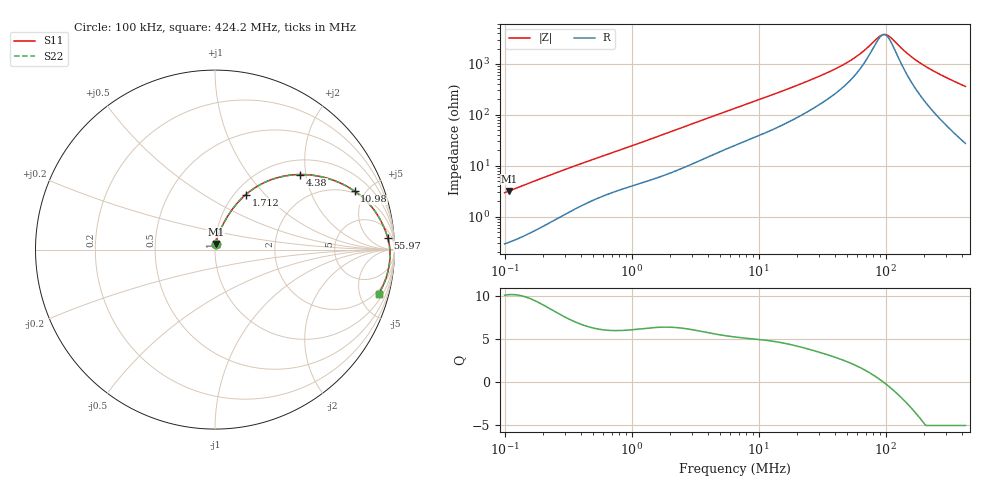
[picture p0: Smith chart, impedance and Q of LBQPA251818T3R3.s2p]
! LBQPA251818T3R3  S-PARAMETER MODEL  ( General Type )
! Model Generated by TAIYO YUDEN Corporation (http://www.ty-top.com)
! Version 1.0
! TAIYO YUDEN Control No. 191025NI43SB-FBB
! Copyright(c) 2019 TAIYO YUDEN CO.,LTD. All Rights Reserved.
! Product Description (link to TY-COMPAS)
! https://ds.yuden.co.jp/TYCOMPAS/or/detail?pn=LBQPA251818T3R3M&u=M
! Products Name : Inductors
! Characteristics :
!  Inductance : 3.3 uH , SRF(min) : 54 MHz , DC Resistance(max) : 0.208 Ohm
!  Rated Current : Saturation :730 mA , Temp Rise : 560 mA (20 degC)
!  Case Size : 2.5 x 1.8 / 0.098 x 0.071 [mm/inch] , Thickness : 1.8 / 0.071 [mm/inch]
!  (Conditions: Temperature = 25 degC , DC Bias Current/Voltage = 0A / 0V)
! External Node Assignments :
!  1  o---GGG---o  2
! GND o---------o GND
! Frequency Range : 0.1MHz  -  424.248007MHz  [ 402 STEP ]
# MHz S RI R 50
! Freq[MHz].  S11 Real  S11 Imag  S21 Real  S21 Imag  S12 Real  S12 Imag  S22 Real  S22 Imag
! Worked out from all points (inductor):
!   401 points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, 100 kHz to 424.2 MHz, reference 50 ohm
!   read as one part in series: L = 4.64 uH near 104.3 kHz
!   highest Q = 10.1 at 108.7 kHz (marker M1), where L = 4.66 uH
!   self-resonance near 96.29 MHz
!   S11 on the Smith chart (normalised r, x): 100 kHz: 1.01, +0.06; 1.712 MHz: 1.12, +0.79; 4.38 MHz: 1.33, +1.85; 10.98 MHz: 1.86, +4.19; 55.97 MHz: 12, +23; 424.2 MHz: 1.55, -7.19
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0.1  0.00375 0.0291  0.9962 -0.0291  0.9962 -0.0291  0.00375 0.0291
0.108712  0.00413 0.0316  0.9959 -0.0316  0.9959 -0.0316  0.00413 0.0316
0.40516  0.0275 0.105  0.9725 -0.105  0.9725 -0.105  0.0275 0.105
0.914785  0.0783 0.1982  0.9217 -0.1982  0.9217 -0.1982  0.0783 0.1982
1.641544  0.1626 0.2987  0.8374 -0.2987  0.8374 -0.2987  0.1626 0.2987
1.711555  0.1714 0.3065  0.8286 -0.3065  0.8286 -0.3065  0.1714 0.3065
2.884808  0.3189 0.3915  0.6811 -0.3915  0.6811 -0.3915  0.3189 0.3915
4.380241  0.4729 0.4182  0.5271 -0.4182  0.5271 -0.4182  0.4729 0.4182
6.650878  0.6267 0.3973  0.3733 -0.3973  0.3733 -0.3973  0.6267 0.3973
10.97833  0.7778 0.3257  0.2222 -0.3257  0.2222 -0.3257  0.7778 0.3257
16.66929  0.8634 0.249  0.1366 -0.249  0.1366 -0.249  0.8634 0.249
26.38981  0.9193 0.1692  0.0807 -0.1692  0.0807 -0.1692  0.9193 0.1692
40.91535  0.9492 0.1054  0.0508 -0.1054  0.0508 -0.1054  0.9492 0.1054
55.96571  0.9624 0.0655  0.0376 -0.0655  0.0376 -0.0655  0.9624 0.0655
67.53726  0.968 0.0427  0.032 -0.0427  0.032 -0.0427  0.968 0.0427
90.47116  0.9735 0.00757  0.0265 -0.00757  0.0265 -0.00757  0.9735 0.00757
98.35271  0.9743 -0.00259  0.0257 0.00259  0.0257 0.00259  0.9743 -0.00259
106.9209  0.9749 -0.0129  0.0251 0.0129  0.0251 0.0129  0.9749 -0.0129
149.337  0.974 -0.0563  0.026 0.0563  0.026 0.0563  0.974 -0.0563
191.8651  0.9693 -0.0928  0.0307 0.0928  0.0307 0.0928  0.9693 -0.0928
279.408  0.953 -0.1574  0.047 0.1574  0.047 0.1574  0.953 -0.1574
424.248  0.9125 -0.247  0.0875 0.247  0.0875 0.247  0.9125 -0.247
